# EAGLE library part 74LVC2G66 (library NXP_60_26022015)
Bilateral switch The 74LVC2G66 is a low-power, low-voltage, high-speed Si-gate CMOS device. The 74LVC2G66 provides two single pole, single-throw analog switch functions. Each switch has two input/output terminals (nY and nZ) and an active HIGH enable input (nE). When nE is LOW, the analog switch is turned off. Schmitt trigger action at the enable inputs makes the circuit tolerant of slower input rise and fall times across the entire VCC range from 1.65 V to 5.5 V. AAL Eindhoven MK
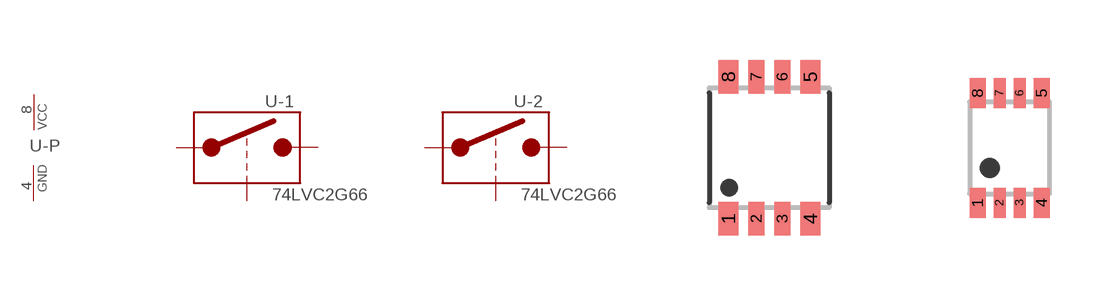
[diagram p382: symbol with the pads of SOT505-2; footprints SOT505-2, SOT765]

Designator prefix U; gates -1=ANALOG_SW_DIG -2=ANALOG_SW_DIG -P=PWRN

## 74LVC2G66DP  [SOT505-2]
1  -1:Y  in
2  -1:Z  out
3  -2:EN  in
4  -P:GND  pwr
5  -2:Y  in
6  -2:Z  out
7  -1:EN  in
8  -P:VCC  pwr

## 74LVC2G66DC  [SOT765]
Pads as for SOT505-2

## 74LVC2G66GT  [SOT833-1]
Pads as for SOT505-2

## 74LVC2G66GD  [SOT996-2/3]
Pads as for SOT505-2

## 74LVC2G66GM  [SOT902-1/2/3]
1  -1:EN  in
2  -2:Z  out
3  -2:Y  in
4  -P:GND  pwr
5  -2:EN  in
6  -1:Z  out
7  -1:Y  in
8  -P:VCC  pwr

## Footprint SOT505-2 (pad centres in mm)
SOT505-2 TSSOP8: plastic thin shrink small outline package; 8 leads; body width 3 mm JEDEC: -- IEC: --
smd 0.5 x 0.85: 1 -1.025,-1.775; 4 1.025,-1.775; 5 1.025,1.775; 8 -1.025,1.775
smd 0.4 x 0.85: 2 -0.325,-1.775; 3 0.325,-1.775; 6 0.325,1.775; 7 -0.325,1.775

## Footprint SOT765 (pad centres in mm)
SOT765 VSSOP8: plastic very thin shrink small outline package; 8 leads; body width 2.3 mm JEDEC: MO-187 IEC: -- JEITA: --
smd 0.4 x 0.75: 1 -0.8,-1.375; 4 0.8,-1.375; 5 0.8,1.375; 8 -0.8,1.375
smd 0.3 x 0.75: 2 -0.25,-1.375; 3 0.25,-1.375; 6 0.25,1.375; 7 -0.25,1.375

## Footprint SOT833-1 (pad centres in mm)
SOT833-1 XSON8: plastic extremely thin small outline package; no leads; 8 terminals; body 1 x 1.95 x 0.5 mm JEDEC: MO-252 IEC: -- JEITA: --
smd 0.3 x 1: 1 -0.775,-0.6
smd 0.25 x 0.95: 2 -0.25,-0.625; 3 0.25,-0.625; 6 0.25,0.625; 7 -0.25,0.625
smd 0.3 x 0.95: 4 0.775,-0.625; 5 0.775,0.625; 8 -0.775,0.625

## Footprint SOT996-2/3 (pad centres in mm)
SOT996-2/3 XSON8U: plastic extremely thin small outline package; no leads;8 terminals; UTLP based; body 3 x 2 x 0.5 mm JEDEC: IEC: -- JEITA: --
smd 0.25 x 1.1: 1 -0.75,-1.45
smd 0.25 x 1: 2 -0.25,-1.5; 3 0.25,-1.5; 4 0.75,-1.5; 5 0.75,1.5; 6 0.25,1.5; 7 -0.25,1.5; 8 -0.75,1.5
